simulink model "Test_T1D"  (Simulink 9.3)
settings: Solver=VariableStepAuto  StartTime=0.0  StopTime=0.5  RelTol=1e-3
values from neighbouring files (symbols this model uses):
  Tstep = 0.000050    (= 5e-05)    [TestOrthOsc_init.m]    (also in Test_PIDctrl_init.m = 0.0001)
libraries: libVishia_Ctrl x2, libVishia_CtrlSfn x1, libVishia_Conv x1

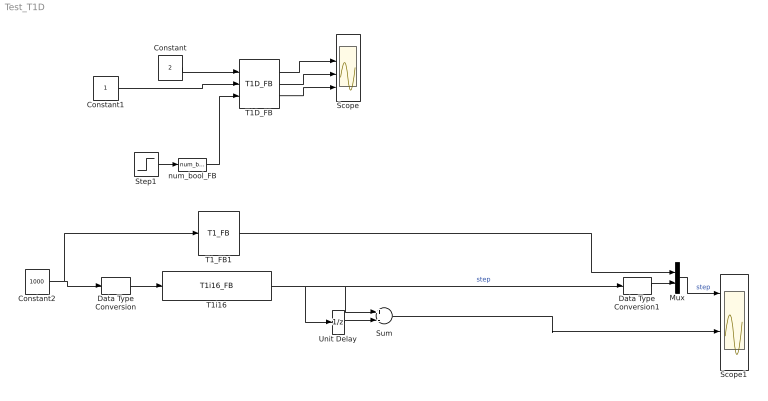
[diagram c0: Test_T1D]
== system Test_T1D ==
  Constant : Constant  Value=2
  Constant1 : Constant
  Constant2 : Constant  Value=1000  OutDataTypeStr=single
  Data Type Conversion : DataTypeConversion  OutDataTypeStr=int16
  Data Type Conversion1 : DataTypeConversion  OutDataTypeStr=single
  Mux : Mux  Inputs=2
  Scope : Scope  NumInputPorts=4
  Scope1 : Scope  NumInputPorts=4
  Step1 : Step  Time=0.1  Before=1  After=0  SampleTime=Tstep
  Sum : Sum  Inputs=+-
  T1D_FB : libVishia_Ctrl/T1D_FB  T1=0.5  y0=0  Tstep=Tstep
  T1_FB1 : libVishia_Ctrl/T1_FB  T1=0.1  y0=0  Tstep=Tstep
  T1i16 : libVishia_CtrlSfn/T1i16_FB  Ts=0.1  Tstep=Tstep
  Unit Delay : UnitDelay  SampleTime=-1  HasFrameUpgradeWarning=on
  num_bool_FB : libVishia_Conv/num_bool_FB  SystemSampleTime=-1
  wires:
  Constant1/1 -> T1D_FB/2
  Constant/1 -> T1D_FB/1
  Step1/1 -> num_bool_FB/1
  num_bool_FB/1 -> T1D_FB/3
  T1D_FB/1 -> Scope/2
  T1D_FB/2 -> Scope/3
  T1D_FB/3 -> Scope/4
  Data Type Conversion/1 -> T1i16/1
  Constant2/1 -> T1_FB1/1, Data Type Conversion/1
  Mux/1 -> Scope1/1  "step"
  T1_FB1/2 -> Mux/1
  T1i16/1 -> Unit Delay/1, Sum/1, Data Type Conversion1/1  "step"
  Data Type Conversion1/1 -> Mux/2
  Unit Delay/1 -> Sum/2
  Sum/1 -> Scope1/3
